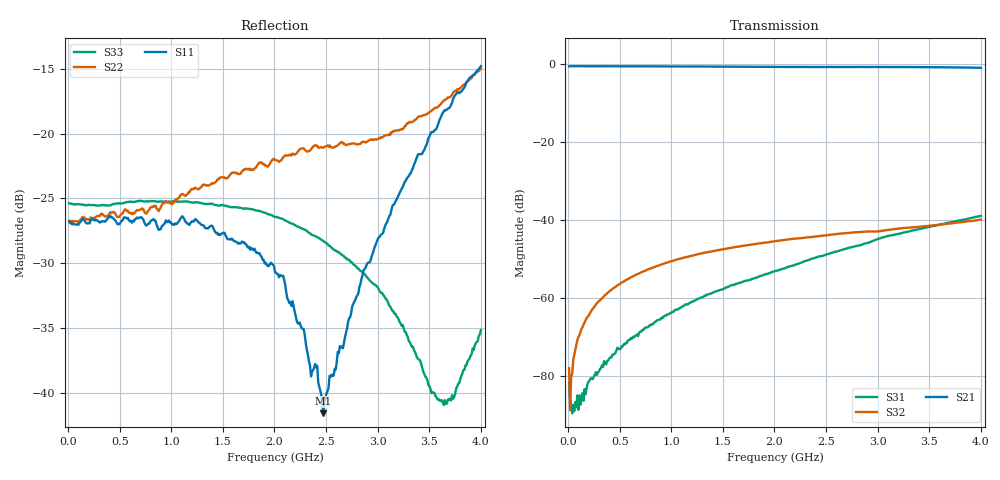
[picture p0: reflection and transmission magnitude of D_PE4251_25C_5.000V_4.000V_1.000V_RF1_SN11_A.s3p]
! Device ID: PE4251_SoldCshunt_081809
! Dir: c:\Test Bench Repositories\Bench_Software_CVI_Version_8\trunk\PSC 4Port_VNA Bench\datalog\4250\TEST\PE4251_SoldCshunt_081809\25C\5p000000\RF1
! Serial: 11
! Insertion: A
! Temp: 25C
! VDD: 5.000
! Control_Hi: 80.000
! Control_Lo: 20.000
! Logic State: RF1
! Port 1: RFC
! Port 2: RF1
! Port 3: RF2
! V1 = 1.00
! V2 = 4.00
! V3 = 1.00
! IDD: 6.296040e-05
! FILE NAME
! DATE 08/18/09  20:14
! CORRECTED  DATA
#  Hz  S  RI  R  50.00
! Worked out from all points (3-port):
!   401 points, 10 MHz to 4 GHz, reference 50 ohm
!   strongest paths, dB at 10 MHz, 1.008 GHz, 2.005 GHz, 3.002 GHz, 4 GHz:
!     S21: -0.6, -0.6, -0.7, -0.7, -1.0
!     S32: -78.1, -50.6, -45.5, -43.0, -39.9
!     S31: -81.9, -63.6, -53.2, -44.9, -39.0
!   lowest |S11| = -41.6 dB at 2.474 GHz (marker M1), VSWR 1.02, Z = 49.9 - j0.832 ohm
!   |S11| at or under -10 dB: start of sweep to end of sweep
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1e7  0.0459 0.000114  0.9381 -0.00353  -1.54e-05 2.37e-05
     0.9376 -0.00379  0.0461 -0.000156  -1.38e-05 -1.23e-05
     7.86e-05 -1.64e-05  0.000124 1.44e-05  0.0539 -0.000573
1.79575e8  0.0451 0.000512  0.9368 -0.0609  -4e-06 -7e-05
           0.9362 -0.0613  0.0467 0.000358  5.37e-05 0.000541
           -3.55e-06 -6.88e-05  5.96e-05 0.000544  0.053 -0.000957
2.6935e8  0.0465 -1.57e-05  0.9335 -0.0881  -2.61e-05 -9.29e-05
          0.9334 -0.0876  0.0478 0.000134  7.19e-05 0.000808
          -3.16e-05 -0.000106  6.88e-05 0.000814  0.0528 -0.00184
4.98775e8  0.0445 -0.00456  0.9209 -0.1655  -0.000139 -0.000169
           0.9214 -0.1646  0.0476 -0.00383  0.000146 0.00149
           -0.000134 -0.000173  0.000151 0.00149  0.0536 -0.00489
1.197025e9  0.0436 -0.0142  0.8508 -0.3784  -0.000844 -0.000255
            0.8513 -0.3772  0.0586 -0.0171  0.000623 0.0034
            -0.000845 -0.000255  0.000606 0.0034  0.0539 -0.00676
2.005e9  0.0263 -0.0128  0.7162 -0.5786  -0.00219 -0.000161
         0.7162 -0.5793  0.0689 -0.0387  0.00109 0.0052
         -0.00219 -0.000161  0.0011 0.00521  0.0476 -0.00416
2.473825e9  -0.000469 -0.00832  0.6222 -0.6748  -0.00349 -0.000164
            0.6195 -0.6738  0.0632 -0.0615  0.00121 0.00613
            -0.00347 -0.00016  0.0012 0.00617  0.0386 -5.18e-05
2.872825e9  -0.0197 -0.0226  0.529 -0.7503  -0.00494 1.91e-05
            0.5317 -0.7478  0.0429 -0.0825  0.00125 0.00692
            -0.00496 2.74e-05  0.00126 0.00693  0.0286 0.00276
3.62095e9  -0.0984 -0.0654  0.3142 -0.8525  -0.00861 0.00169
           0.3156 -0.8535  -0.0456 -0.1234  0.000293 0.00869
           -0.00863 0.00169  0.00029 0.00871  0.00233 0.00908
4e9  -0.1637 -0.0798  0.1816 -0.8789  -0.0108 0.0031
     0.1811 -0.876  -0.1255 -0.1274  -0.000397 0.01
     -0.0108 0.00307  -0.000442 0.0101  -0.0138 0.0107
